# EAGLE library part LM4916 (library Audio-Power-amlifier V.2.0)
LM4916 1.5V, Mono 85mW BTL Output, 14mW Stereo Headphone Audio Amplifier
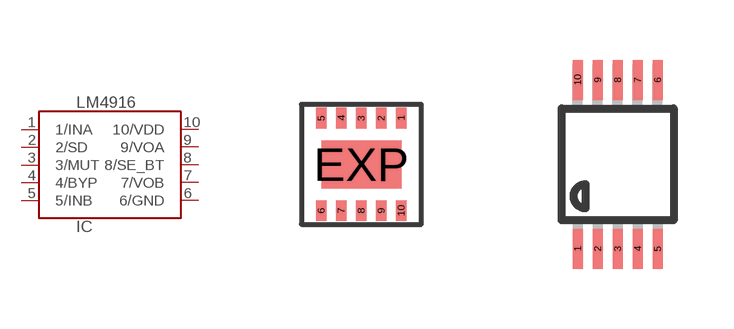
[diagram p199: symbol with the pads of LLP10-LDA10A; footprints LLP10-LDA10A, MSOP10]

Designator prefix IC

## LM4916LM4916LD  [LLP10-LDA10A]
1  1/INA  in
2  2/SD
3  3/MUT  in
4  4/BYP  in
5  5/INB  in
6  6/GND  pwr
7  7/VOB  out
8  8/SE_BT
9  9/VOA  out
10  10/VDD  pwr

## LM4916LM4916MM  [MSOP10]
Pads as for LLP10-LDA10A

## Footprint LLP10-LDA10A (pad centres in mm)
LLP10-LDA10A_3x3 body www.national.com
smd 0.26 x 0.52: 1 1,1.16; 2 0.5,1.16; 3 0,1.16; 4 -0.5,1.16; 5 -1,1.16; 6 -1,-1.16; 7 -0.5,-1.16; 8 0,-1.16; 9 0.5,-1.16; 10 1,-1.16
smd 2 x 1.2: EXP 0,0

## Footprint MSOP10 (pad centres in mm)
10-Lead Mini Small Outline Package [MSOP] MUB10A www.national.com
smd 0.25 x 1: 1 -1,-2.113; 2 -0.5,-2.113; 3 0,-2.113; 4 0.5,-2.113; 5 1,-2.113; 6 1,2.113; 7 0.5,2.113; 8 0,2.113; 9 -0.5,2.113; 10 -1,2.113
